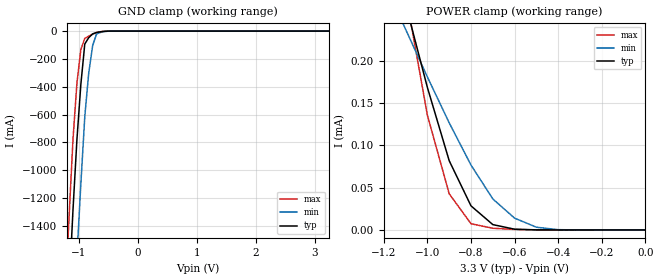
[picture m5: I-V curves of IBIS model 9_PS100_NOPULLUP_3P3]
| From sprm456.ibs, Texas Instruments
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|   Model Cell 9_PS100_NOPULLUP_3P3
|IDG09_PS100_NOPULLUP_3P3
[Model]   9_PS100_NOPULLUP_3P3
Model_type   Input
Polarity   Non-Inverting
Vinl =  0.8V
Vinh =  2V
C_comp   1.447p   1.213p   1.874p
[Model Spec]
Vinl   0.8V   0.8V   0.8V
Vinh   2V   2V   2V
[Temperature Range]   25   125   -40
[Voltage Range]   3.3   3   3.6
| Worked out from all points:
|   GND clamp passes 1 mA (typ) near -0.53 V on its own axis
|   POWER clamp passes 1 mA (typ) near -1.78 V on its own axis
[POWER_clamp]
|   voltage   I(typ)   I(min)   I(max)
-3.3V     2.695mA    1.572mA    4.067mA
-1.1V     266.9uA    237.2uA    279.9uA
-1.067V   234.1uA    218.4uA    231.7uA
-1V       168.4uA    180.8uA    135.5uA
-900mV    81.82uA    126.6uA    42.76uA
-800mV    28.47uA    76.69uA    7.358uA
-700mV    6.356uA    36.66uA    2.023uA
-600mV    884.9nA    13.95uA    630.3nA
-500mV    144.6nA    3.256uA    75.42nA
-400mV    11.27nA    351.3nA    2.764nA
0V        62.11pA    8.891nA    697.2fA
[GND_clamp]
|   voltage   I(typ)   I(min)   I(max)
-3.3V     -22.54A    -23.36A    -22.09A
-1.233V   -2.454A    -3.359A    -1.924A
-1.167V   -1.863A    -2.762A    -1.341A
-1.1V     -1.287A    -2.174A    -780.3mA
-1.033V   -782.2mA   -1.619A    -375.5mA
-966.7mV  -384.1mA   -1.1A      -132.9mA
-900mV    -92.98mA   -616.1mA   -52.34mA
-833.3mV  -47.56mA   -302.3mA   -36.12mA
-766.7mV  -19.98mA   -103.7mA   -22.14mA
-700mV    -10.23mA   -20.37mA   -10.41mA
-500mV    -282.6uA   -891uA     -99.21uA
3.233V    60.54pA    18.5nA     577.3fA
